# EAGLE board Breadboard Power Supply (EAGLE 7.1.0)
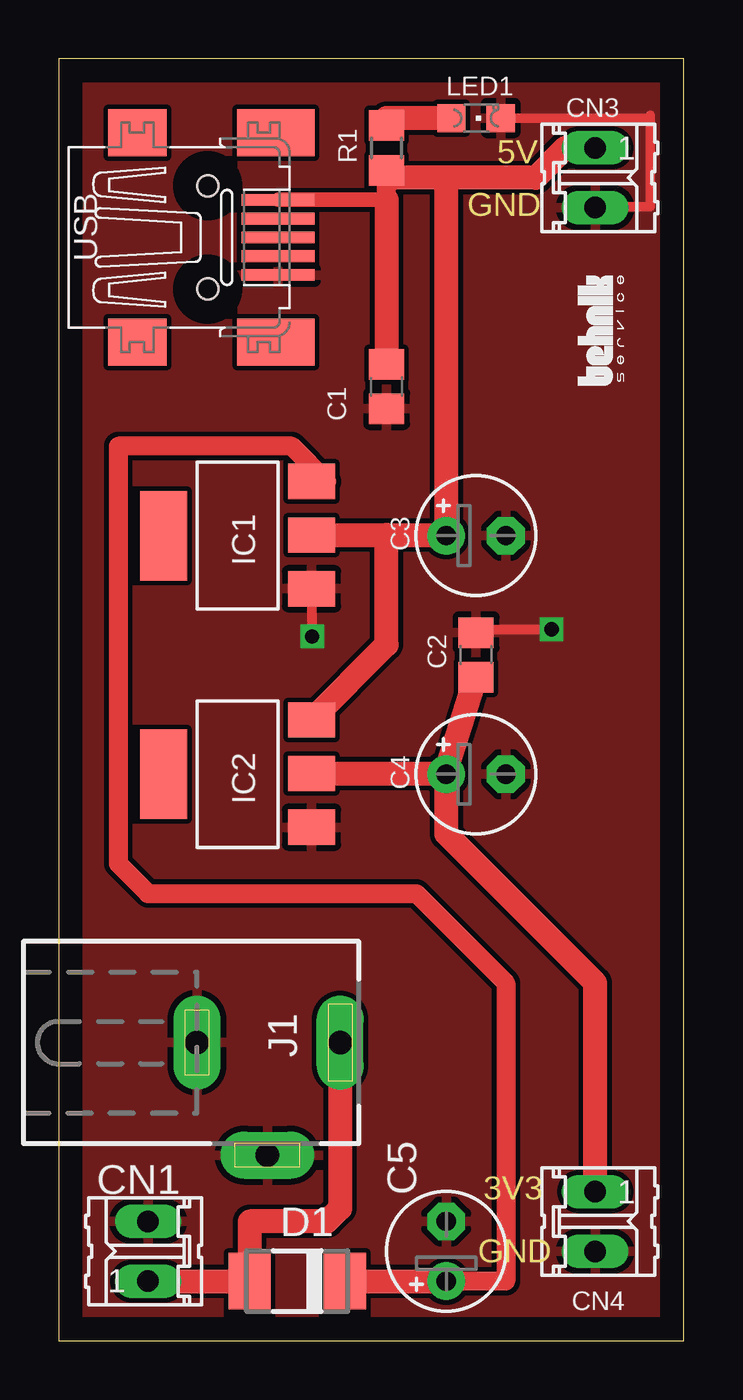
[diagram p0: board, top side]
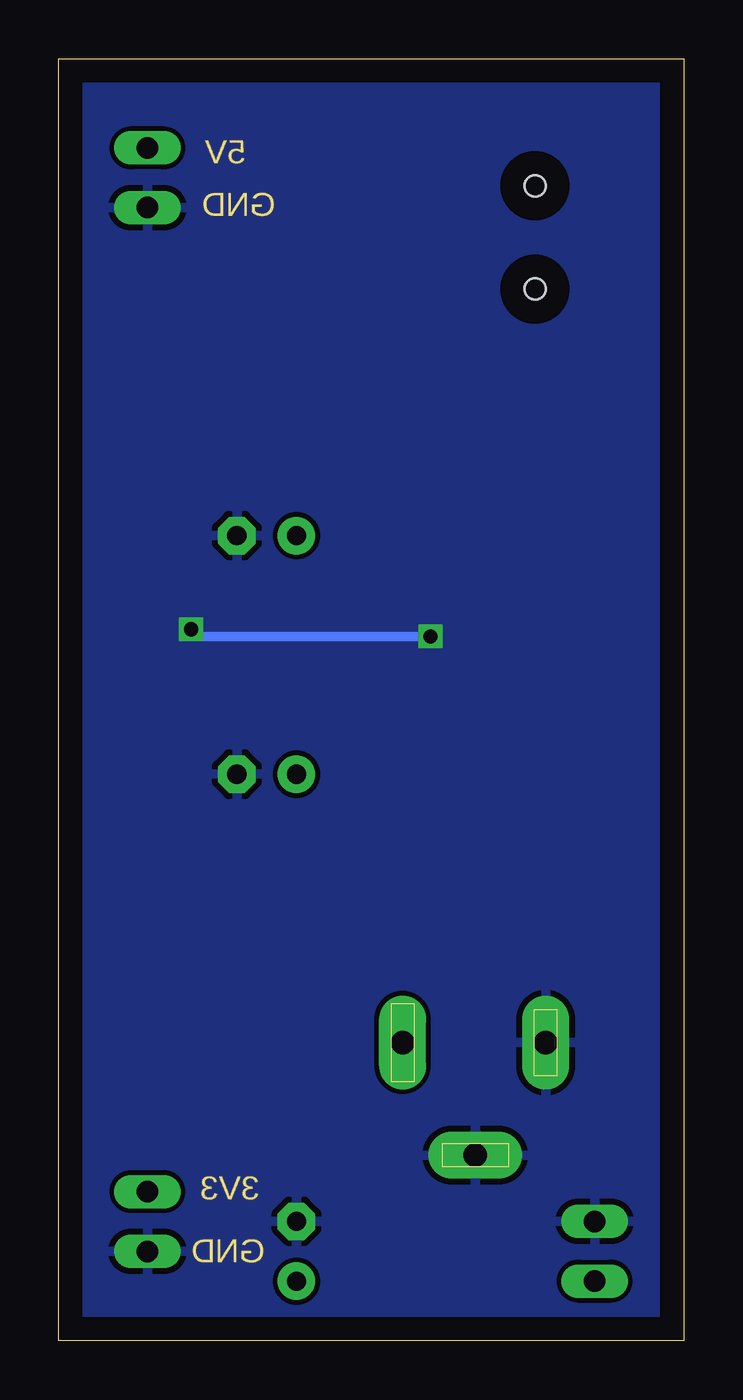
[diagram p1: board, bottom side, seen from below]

Size 26.64 x 54.6 mm. Coordinates in mm from the lower left corner, seen from the top.
Outline: 0,0 26.64,0 26.64,54.6 0,54.6 0,0
Copper layers (1*16): Top 0.035mm / dielectric 1.5mm / Bottom 0.035mm
Design rules "default": minimum track width 10mil, minimum drill 24mil, track to track 8mil, track to pad 8mil, pad to pad 8mil, via to via 8mil, smd to smd 8mil, copper to edge 40mil, drill to drill 8mil, minimum pad ring 10mil, minimum via ring 8mil, stop-mask expansion 4mil, vias tented up to drill 0mil, thermal gap 10mil

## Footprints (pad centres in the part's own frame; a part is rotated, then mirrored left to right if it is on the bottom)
C0805 = smd 1.3 x 1.5: 1 -0.95,0; 2 0.95,0
E2,5-5 = drill 0.813 pad 1.6: + -1.27,0 | drill 0.813 pad 1.6 octagon: - 1.27,0
02P = drill 0.914 long: 1 -1.27,0; 2 1.27,0
DO-214AC = smd 1.8 x 2.4: A 2.025,0; C -2.025,0
SOT223 = smd 1.499 x 2.007: 1 -2.261,-3.15; 2 0.025,-3.15; 3 2.311,-3.15 | smd 3.81 x 2.007: 4 0,3.15
DCJ0202 = drill 1 pad 2 long: 1 0,3.1; 2 4.8,0; 3 0,-3
CHIPLED_0805 = smd 1.2 x 1.2: A 0,-1.05; C 0,1.05
R0805 = smd 1.3 x 1.5: 1 -0.95,0; 2 0.95,0
32005-201 = smd 3.1 x 0.5: 1 3,1.6; 2 3,0.8; 3 3,0; 4 3,-0.8; 5 3,-1.6 | smd 2.5 x 2: M1 -3,-4.45; M2 -3,4.45 | smd 3.3 x 2: M3 2.9,4.45; M4 2.9,-4.45 | hole 0.9: 0,2.2; 0,-2.2

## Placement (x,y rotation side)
C1  100n  [C0805]  13.97,40.64 270 top
C2  100n  [C0805]  17.78,29.21 90 top
C3  22uF  [E2,5-5]  17.78,34.29 0 top
C4  22uF  [E2,5-5]  17.78,24.13 0 top
C5  100uF  [E2,5-5]  16.51,3.81 90 top
CN1  [02P]  3.81,3.81 90 top
CN3  [02P]  22.86,49.53 270 top
CN4  [02P]  22.86,5.08 270 top
D1  M7  [DO-214AC]  10.16,2.54 180 top
IC1  1117-5  [SOT223]  7.62,34.29 90 top
IC2  1117-3.3  [SOT223]  7.62,24.13 90 top
J1  DCIN  [DCJ0202]  8.89,12.7 270 top
LED1  [CHIPLED_0805]  17.78,52.07 270 top
R1  [R0805]  13.97,50.8 90 top
U$1  [LOGOT]  24.13,40.64 90 top
USB  MINI-USB  [32005-201]  6.35,46.99 0 top

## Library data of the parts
C1-C5 R1 = rcl
CN1 CN3 CN4 = con-amp-quick; OC_FARNELL: unknown; OC_NEWARK: unknown
D1 = diode
IC1 IC2 = burr-brown; MPN: REG1117; OC_FARNELL: 1097566; OC_NEWARK: 14P6981
J1 = con-jack; OC_FARNELL: unknown; OC_NEWARK: unknown
LED1 = led
U$1 = logoo
USB = con-cypressindustries; OC_FARNELL: unknown; OC_NEWARK: unknown

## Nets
+3V3: C2.1 C4.+ CN4.1 IC2.2
DCIN: C5.+ D1.C IC1.3
GND: C1.2 C2.2 C3.- C4.- C5.- CN1.2 CN3.2 CN4.2 IC1.1 IC2.1 J1.2 J1.3 LED1.C USB.5
N$1: LED1.A R1.2
N$2: CN1.1 D1.A J1.1
VCC: C1.1 C3.+ CN3.1 IC1.2 IC2.3 R1.1 USB.1

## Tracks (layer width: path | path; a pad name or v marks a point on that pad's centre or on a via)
+3V3
  Top 1.016: IC2.2 16.48,24.16 | 16.48,24.16 C4.+ 16.51,21.59 22.86,15.24 CN4.1 | 16.48,24.16 C2.1
DCIN
  Top 0.813: IC1.3 11.43,36.6 9.93,38.1 2.54,38.1 2.54,20.32 3.81,19.05 15.24,19.05 19.05,15.24 19.05,2.54 C5.+
  Top 1.016: D1.C C5.+
GND  (via drill 0.6)
  Top 0.406: IC1.1 10.8,32.03 v10.8,30 | v21,30.3 17.78,30.3 C2.2 | LED1.C 25.2,52.07 | 25.2,52.07 25.2,52.2 | 25.2,52.07 25.2,48.3 22.86,48.3 CN3.2
  Bottom 0.406: v10.8,30 21,30 v21,30.3
  pour Top: 0,54.61 26.67,54.61 26.67,0 0,0
  pour Bottom: 0,54.6 26.7,54.6 26.7,0 0,0
N$1
  Top 1.016: LED1.A 13.97,52.07 R1.2
N$2
  Top 1.016: CN1.1 D1.A 8.13,5.08 11.43,5.08 11.99,5.64 J1.1
VCC
  Top 0.61: USB.1 13.97,48.59
  Top 0.813: 13.97,48.59 R1.1
  Top 1.016: 13.97,48.59 C1.1 | CN3.1 21.59,50.8 20.32,49.53 16.51,49.53 | 16.51,49.53 14.29,49.53 R1.1 | IC1.2 13.97,34.31 | 13.97,34.31 16.48,34.31 | 16.48,34.31 C3.+ | 16.48,34.31 16.51,34.31 16.51,49.53 | IC2.3 13.97,29.64 13.97,34.31

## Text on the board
Dimension: 5V | GND | 3V3 | GND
